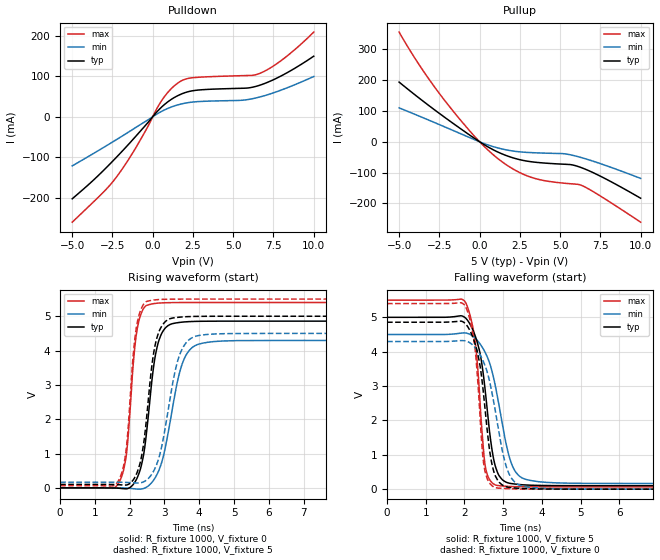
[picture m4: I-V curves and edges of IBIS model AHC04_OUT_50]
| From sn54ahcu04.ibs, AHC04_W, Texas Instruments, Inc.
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[Model]   AHC04_OUT_50
Model_type  Output
Vref =   0
Rref =   1000
Cref =   50p
Vmeas =   2.5
| variable   typ   min   max
C_comp   2.64pF   1.48pF   3.62pF
| C_pullup   2.78pF   1.48pF   3.62pF
| C_pulldown   2.50pF   1.75pF   3.39pF
[Temperature Range]   40   100   -40
| Ambient temperature   25   85   -40
[Voltage range]   5   4.5   5.5
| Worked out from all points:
|   slope of the pulldown table from 0 to 0.75 V, typ, clamps not added: 24.2 ohm
|   slope of the pullup table from 0 to 0.75 V, typ, clamps not added: 32.1 ohm
|   rising waveform, R_fixture 1000, V_fixture 0: 20-80 % time 342ps typ, 503ps min, 254ps max; typ from 0 V to 4.86 V
|   falling waveform, R_fixture 1000, V_fixture 5: 20-80 % time 332ps typ, 476ps min, 228ps max; typ from 5 V to 0.101 V
|   rising waveform, R_fixture 1000, V_fixture 5: 20-80 % time 336ps typ, 481ps min, 253ps max; typ from 0.101 V to 5 V
|   falling waveform, R_fixture 1000, V_fixture 0: 20-80 % time 319ps typ, 451ps min, 218ps max; typ from 4.86 V to 0 V
[Pulldown]
| AHC04_OUT_50
|   Voltage   I(typ)   I(min)   I(max)
-5V       -203.2mA   -121.7mA   -261.1mA
-3.07V    -133.5mA   -76.46mA   -187mA
-2.27V    -101mA     -57.05mA   -150.2mA
-1.02V    -46.97mA   -25.75mA   -74.62mA
510mV     22.36mA    12.39mA    37.2mA
970mV     37.83mA    21.14mA    61.73mA
1.46V     50.19mA    28.2mA     80.49mA
2.405V    63.82mA    36.03mA    96.15mA
5.545V    70.46mA    40.77mA    101.7mA
6.605V    77.49mA    48.42mA    106.7mA
8.09V     103.5mA    67.7mA     142.5mA
10V       149.9mA    99.56mA    209.6mA
[Pullup]
| AHC04_OUT_50
|   Voltage   I(typ)   I(min)   I(max)
-5V       193.4mA    109.9mA    355.5mA
-3.6V     135.3mA    79.82mA    237.4mA
-2.035V   74.16mA    45.29mA    124.9mA
-215mV    7.5mA      4.696mA    11.93mA
1.165V    -34.04mA   -20.45mA   -55.72mA
2.21V     -54.21mA   -30.99mA   -92.25mA
3.26V     -65.13mA   -35.31mA   -116.2mA
4.09V     -69.26mA   -36.91mA   -126.6mA
5.215V    -72.73mA   -38.72mA   -134.1mA
6.085V    -79.6mA    -47.92mA   -137.9mA
7.11V     -101.6mA   -64.04mA   -163.3mA
10V       -183mA     -118.8mA   -260.7mA
[Ramp]
| AHC04_OUT_50
| variable   typ   min   max
dV/dt_r   2.93/3.50E-10   2.60/5.11E-10   3.25/2.61E-10
dV/dt_f   2.97/3.43E-10   2.63/4.86E-10   3.28/2.32E-10
R_load = 1000
[Rising Waveform]
| AHC04_OUT_50
R_fixture =   1000
C_fixture =   0
L_fixture =   0
V_fixture =   0
V_fixture_min = 0
V_fixture_max = 0
|   Time   V(typ)   V(min)   V(max)
0s        1.078nV    1.79nV     663.1pV
1.7ns     -12.1mV    79.96uV    169.9mV
1.905ns   -27.78mV   -6.768mV   965.3mV
2.115ns   116.6mV    -25.49mV   3.755V
2.23ns    326.7mV    -36.21mV   4.705V
2.42ns    1.093V     -10.96mV   5.256V
2.775ns   4.044V     371.6mV    5.378V
3.565ns   4.833V     3.754V     5.399V
4.45ns    4.856V     4.264V     5.4V
50ns      4.857V     4.295V     5.4V
[Falling Waveform]
| AHC04_OUT_50
R_fixture =   1000
C_fixture =   0
L_fixture =   0
V_fixture =   5
V_fixture_min = 4.5
V_fixture_max = 5.5
|   Time   V(typ)   V(min)   V(max)
0s        5V         4.5V       5.5V
2.015ns   4.992V     4.546V     5.458V
2.27ns    4.48V      4.4V       4.351V
2.415ns   3.876V     4.206V     2.279V
2.55ns    2.715V     3.943V     590.2mV
2.735ns   982.3mV    3.32V      164.9mV
2.92ns    351.8mV    2.265V     97.36mV
3.33ns    145.7mV    487.4mV    73.16mV
4.32ns    104.1mV    185.4mV    65.91mV
50ns      100.8mV    165mV      65.08mV
[Rising Waveform]
| AHC04_OUT_50
R_fixture =   1000
C_fixture =   0
L_fixture =   0
V_fixture =   5
V_fixture_min = 4.5
V_fixture_max = 5.5
|   Time   V(typ)   V(min)   V(max)
0s        100.8mV    165mV      65.08mV
1.69ns    91.27mV    164.8mV    234.3mV
1.905ns   83.27mV    158.7mV    1.165V
2.095ns   223.3mV    146.8mV    3.805V
2.215ns   453.8mV    141.5mV    4.805V
2.4ns     1.284V     176.2mV    5.35V
2.73ns    4.154V     572.6mV    5.476V
3.455ns   4.974V     3.923V     5.499V
4.23ns    4.998V     4.47V      5.5V
50ns      5V         4.5V       5.5V
[Falling Waveform]
| AHC04_OUT_50
R_fixture =   1000
C_fixture =   0
L_fixture =   0
V_fixture =   0
V_fixture_min = 0
V_fixture_max = 0
|   Time   V(typ)   V(min)   V(max)
0s        4.857V     4.295V     5.4V
2.01ns    4.83V      4.318V     5.351V
2.265ns   4.261V     4.132V     4.175V
2.405ns   3.568V     3.902V     2.052V
2.515ns   2.517V     3.639V     603.5mV
2.68ns    903.9mV    2.976V     133.9mV
2.865ns   244.7mV    1.825V     31.07mV
3.23ns    42.02mV    293.2mV    10.01mV
4.17ns    3.592mV    17.46mV    1.133mV
50ns      -7.167nV   -17.22nV   -3.843nV
